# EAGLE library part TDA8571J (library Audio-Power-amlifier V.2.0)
2x40W Stereo BTL Amplifier
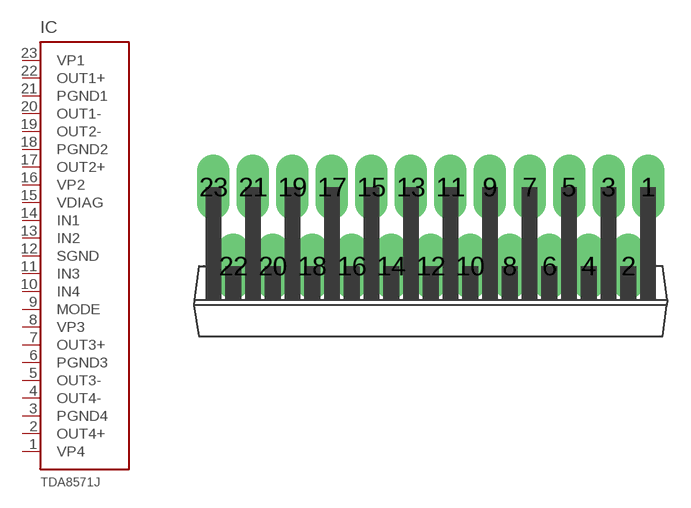
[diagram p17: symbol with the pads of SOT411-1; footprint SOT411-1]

Designator prefix IC

## TDA8571J  [SOT411-1]
1  VP4  pwr
2  OUT4+  out
3  PGND4  pwr
4  OUT4-  out
5  OUT3-  out
6  PGND3  pwr
7  OUT3+  out
8  VP3  pwr
9  MODE
10  IN4  in
11  IN3  in
12  SGND  pwr
13  IN2  in
14  IN1  in
15  VDIAG
16  VP2  pwr
17  OUT2+  out
18  PGND2  pwr
19  OUT2-  out
20  OUT1-  out
21  PGND1  pwr
22  OUT1+  out
23  VP1  pwr

## Footprint SOT411-1 (pad centres in mm)
drill 1.4 long: 1 13.97,5.08; 2 12.7,0; 3 11.43,5.08; 4 10.16,0; 5 8.89,5.08; 6 7.62,0; 7 6.35,5.08; 8 5.08,0; 9 3.81,5.08; 10 2.54,0; 11 1.27,5.08; 12 0,0; 13 -1.27,5.08; 14 -2.54,0; 15 -3.81,5.08; 16 -5.08,0; 17 -6.35,5.08; 18 -7.62,0; 19 -8.89,5.08; 20 -10.16,0; 21 -11.43,5.08; 22 -12.7,0; 23 -13.97,5.08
